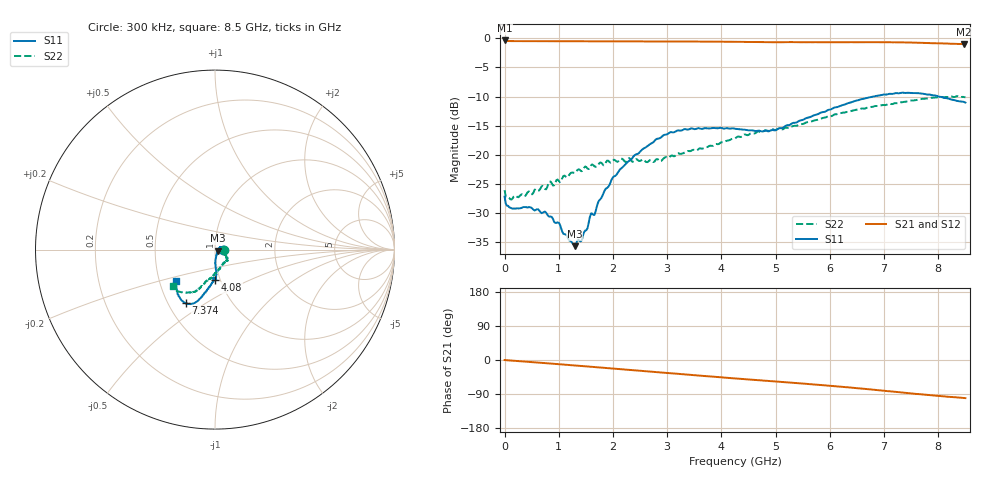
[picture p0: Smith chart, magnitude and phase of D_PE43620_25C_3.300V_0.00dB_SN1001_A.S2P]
! device id: pe43620
! dir: c:\dsa\pe43620\data\pe43620\025c\3p300v\00p00db
! Serial: 1001
! Insertion: A
! Temp: 25C
! VDD: 3.300V
! Attenuation Step: 0.00dB
! IDD: 8.983917e-03mA
! FILE NAME
! DATE 10-22-2008 14:03:40
! CORRECTED  DATA
#  Hz  S  RI  R  50.00
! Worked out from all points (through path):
!   401 points, 300 kHz to 8.5 GHz, reference 50 ohm
!   highest |S21| = -0.36 dB at 300 kHz (marker M1); lowest = -1.0 dB at 8.479 GHz (marker M2)
!   group delay of S21, straight-line fit = 32.6 ps
!   lowest |S11| = -35.6 dB at 1.297 GHz (marker M3), VSWR 1.03, Z = 51.6 - j0.614 ohm
!   |S11| at or under -10 dB: start of sweep to 6.796 GHz; 8.018 GHz to end of sweep
!   |S22| runs from -27.6 to -9.9 dB; largest |S21 - S12| = 0.0053
!   S11 on the Smith chart (normalised r, x): 300 kHz: 1.09, -0.00; 4.08 GHz: 0.95, -0.33; 7.374 GHz: 0.61, -0.41; 8.5 GHz: 0.61, -0.23
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300000  0.0439 -0.000493  0.959 -0.00275  0.9548 -0.00236  0.0499 -0.000758
1.065463e8  0.0352 0.00224  0.9467 -0.0211  0.9474 -0.0212  0.0415 -0.00371
4.465343e8  0.0332 0.0132  0.9423 -0.0814  0.9429 -0.0813  0.0479 -0.00826
7.65273e8  0.029 0.0136  0.9348 -0.1388  0.9352 -0.1395  0.0477 -0.0172
9.990148e8  0.0245 0.00919  0.9275 -0.1807  0.9278 -0.1814  0.0552 -0.0237
1.105261e9  0.0209 0.000912  0.9228 -0.2007  0.9238 -0.2004  0.0589 -0.0308
1.296504e9  0.0154 -0.00596  0.9145 -0.235  0.9148 -0.2356  0.0608 -0.0349
1.424e9  0.0126 -0.0136  0.9076 -0.2589  0.9083 -0.259  0.0625 -0.0369
1.593994e9  0.00909 -0.0301  0.8983 -0.2889  0.899 -0.2901  0.0675 -0.0456
1.99773e9  0.00221 -0.0643  0.8708 -0.3619  0.8725 -0.3613  0.0701 -0.0559
2.401465e9  0.00362 -0.0997  0.8372 -0.4325  0.8376 -0.4326  0.0655 -0.0633
2.8477e9  0.00897 -0.138  0.7949 -0.5056  0.7954 -0.5052  0.0464 -0.0767
3.315183e9  0.00351 -0.1663  0.7418 -0.5775  0.7419 -0.5777  0.03 -0.1003
4.080156e9  0.000679 -0.1694  0.6408 -0.6809  0.6412 -0.6814  0.00036 -0.1315
4.25015e9  -0.00166 -0.1677  0.6165 -0.6998  0.6164 -0.7002  -0.00568 -0.1388
4.972625e9  -0.00525 -0.1625  0.5132 -0.7706  0.5101 -0.7713  -0.0284 -0.1615
5.67385e9  -0.0359 -0.2122  0.4024 -0.8334  0.4033 -0.8349  -0.0585 -0.1856
6.481321e9  -0.0884 -0.2784  0.2537 -0.8916  0.2566 -0.8929  -0.0958 -0.2244
7.09755e9  -0.1387 -0.3041  0.122 -0.919  0.1197 -0.9191  -0.1316 -0.242
7.37379e9  -0.1632 -0.2988  0.0594 -0.9205  0.057 -0.9212  -0.1549 -0.2395
8.478751e9  -0.2202 -0.1799  -0.1608 -0.879  -0.1609 -0.8809  -0.2361 -0.206
8.5e9  -0.2185 -0.1769  -0.1636 -0.8792  -0.1655 -0.8799  -0.2355 -0.2049
